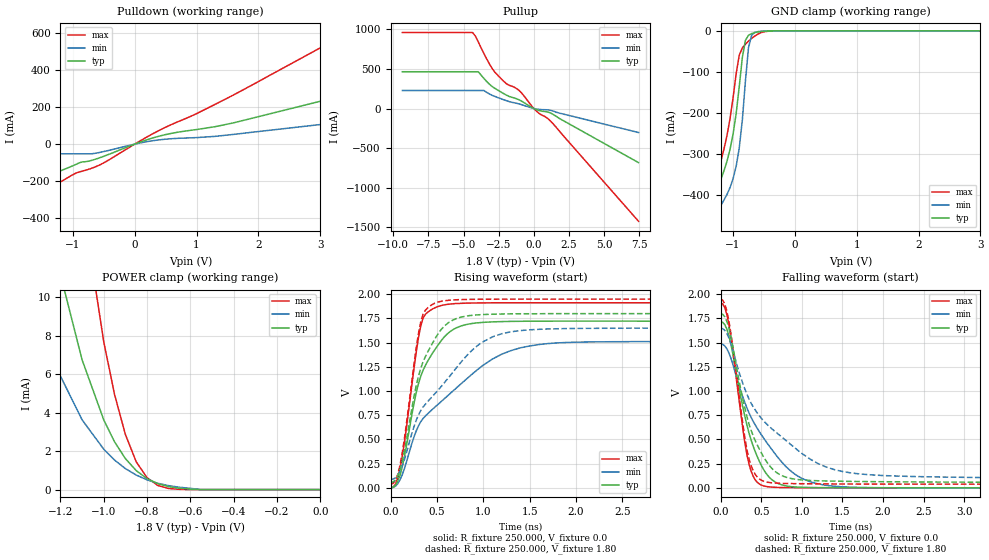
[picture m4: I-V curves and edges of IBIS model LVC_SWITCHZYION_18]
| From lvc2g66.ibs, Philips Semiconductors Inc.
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|   Model LVC_SWITCHZYION_18
[Model]   LVC_SWITCHZYION_18
Model_type   I/O
Polarity   Non-Inverting
Enable   Active-High
Vinl  =  0.63V
Vinh  =  1.17V
Vmeas =  0.90V
Cref  =  30.0pF
Rref  =  1.0k
Vref  =  0.0V
C_comp   7.87pF   4.23pF   10.52pF
[Model Spec]
| Note: The input and output voltage ratings may be exceeded if the input and
|   output current ratings are observed (please refer to the data sheet)
|   Subparameter   typ   min   max
| Thresholds
Vinh   1.17   1.0725   1.2675
Vinl   0.63   0.5775   0.6825
| Overshoot
S_overshoot_high   6.5   6.5   6.5   | Static overshoot
S_overshoot_low   -0.5   -0.5   -0.5
D_overshoot_high   7.2   7.2   7.2   | Dynamic overshoot
D_overshoot_low   -0.95   -0.9   -1.0
D_overshoot_time   3n   3n   3n
| Timing Thresholds
Vmeas   0.9   0.825   0.975
|Ambient temperature:   25   85   -40
[Temperature Range]   25   85   -40
[Voltage Range]   1.80V   1.65V   1.95V
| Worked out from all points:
|   slope of the pulldown table from 0 to 0.27 V, typ, clamps not added: 8.71 ohm
|   slope of the pullup table from 0 to 0.27 V, typ, clamps not added: 13.9 ohm
|   GND clamp passes 1 mA (typ) near -0.50 V on its own axis
|   POWER clamp passes 1 mA (typ) near -0.85 V on its own axis
|   rising waveform, R_fixture 250.000, V_fixture 0.0: 20-80 % time 288ps typ, 734ps min, 161ps max; typ from 0 V to 1.72 V
|   rising waveform, R_fixture 250.000, V_fixture 1.80: 20-80 % time 273ps typ, 613ps min, 161ps max; typ from 0.056 V to 1.8 V
|   falling waveform, R_fixture 250.000, V_fixture 0.0: 20-80 % time 289ps typ, 542ps min, 185ps max; typ from 1.72 V to 0 V
|   falling waveform, R_fixture 250.000, V_fixture 1.80: 20-80 % time 322ps typ, 754ps min, 188ps max; typ from 1.8 V to 0.056 V
|Process Range   nominal   slow   fast
[Pulldown]
| voltage   I(typ)   I(min)   I(max)
-5.5V     -260.6mA   -52.23mA   -443.6mA
-2.3V     -260.6mA   -52.23mA   -443.6mA
-2.1V     -260.6mA   -52.23mA   -388.5mA
-1.05V    -124.3mA   -52.23mA   -175mA
-700mV    -88.32mA   -52.23mA   -131.2mA
400mV     43.47mA    23.26mA    74.9mA
1.6V      115.3mA    52.71mA    266.4mA
3.4V      265.4mA    121.1mA    593.8mA
3.7V      290.4mA    132.4mA    648.5mA
7.6V      615.6mA    279.8mA    1.359A
7.9V      640.6mA    291.2mA    1.414A
11V       899.1mA    408.3mA    1.978A
[Pullup]
| voltage   I(typ)   I(min)   I(max)
-9.35V    464.7mA    227.8mA    959.7mA
-4.35V    464.7mA    227.8mA    959.7mA
-4.15V    464.7mA    227.8mA    913.3mA
-3.95V    464.7mA    227.8mA    840.9mA
-3.55V    380.5mA    227.8mA    695.7mA
-3.15V    306mA      183.2mA    560.8mA
-2.75V    252.5mA    151.3mA    454.6mA
-1.95V    169.5mA    98.93mA    313.6mA
-950mV    101.1mA    53.15mA    212.3mA
200mV     -15.4mA    -7.129mA   -36.04mA
1.2V      -57.74mA   -23.05mA   -160.2mA
7.45V     -683.5mA   -303.4mA   -1.425A
[GND_clamp]
| voltage   I(typ)   I(min)   I(max)
-5.5V     -5.537A    -5.177A    -6.202A
-1.4V     -516.4mA   -571.8mA   -481.4mA
-1.35V    -470.1mA   -525.9mA   -434.4mA
-1.3V     -425.7mA   -482.2mA   -389mA
-1.1V     -319.2mA   -399.7mA   -256.6mA
-950mV    -201.8mA   -330.3mA   -104.7mA
-900mV    -136.1mA   -285.8mA   -59.42mA
-850mV    -65.02mA   -217.8mA   -41.68mA
-800mV    -23.2mA    -121.8mA   -32.63mA
-750mV    -10.8mA    -40.76mA   -25.13mA
-650mV    -4.467mA   -3.964mA   -12.76mA
5.5V      399.8pA    5.379nA    29.89pA
[POWER_clamp]
| voltage   I(typ)   I(min)   I(max)
-9.35V    7.563A     7.588A     7.618A
-1.4V     22.03mA    13.31mA    49.14mA
-1.25V    13.39mA    7.034mA    30.13mA
-1.1V     6.742mA    3.623mA    15.03mA
-1V       3.622mA    2.099mA    7.68mA
-950mV    2.481mA    1.535mA    4.939mA
-900mV    1.612mA    1.092mA    2.864mA
-850mV    987.7uA    755.2uA    1.448mA
-800mV    570.3uA    507.7uA    617.9uA
-750mV    307.3uA    328.4uA    212.9uA
-650mV    69.44uA    121.7uA    13.64uA
0V        0A         0A         0A
[Ramp]
| variable   typ   min   max
dV/dt_r   1.032V/287.683ps   903.161mV/733.821ps   1.147V/161.267ps
dV/dt_f   1.047V/321.661ps   936.914mV/753.761ps   1.147V/187.763ps
R_load = 250.000
[Rising Waveform]
R_fixture   = 250.000
V_fixture   = 0.0
V_fixture_min = 0.0
V_fixture_max = 0.0
| time   V(typ)   V(min)   V(max)
0s        0V         -83.19pV   0V
75ps      61.63mV    39.82mV    93.82mV
125ps     213.7mV    133.3mV    316.6mV
325ps     1.152V     682.8mV    1.672V
375ps     1.264V     741.9mV    1.793V
550ps     1.526V     895.6mV    1.885V
750ps     1.669V     1.067V     1.906V
1.1ns     1.715V     1.332V     1.912V
1.7ns     1.722V     1.491V     1.912V
8.8ns     1.719V     1.505V     1.911V
[Rising Waveform]
R_fixture   = 250.000
V_fixture   = 1.80
V_fixture_min = 1.65
V_fixture_max = 1.95
| time   V(typ)   V(min)   V(max)
0s        55.63mV    86.4mV     38.05mV
50ps      78.77mV    102.3mV    72.84mV
100ps     182.6mV    167.9mV    227.6mV
325ps     1.234V     798.3mV    1.714V
375ps     1.355V     863.8mV    1.835V
525ps     1.61V      1.024V     1.923V
700ps     1.746V     1.229V     1.943V
975ps     1.79V      1.496V     1.949V
1.5ns     1.799V     1.633V     1.95V
8.8ns     1.8V       1.651V     1.95V
[Falling Waveform]
R_fixture   = 250.000
V_fixture   = 0.0
V_fixture_min = 0.0
V_fixture_max = 0.0
| time   V(typ)   V(min)   V(max)
0s        1.717V     1.488V     1.911V
100ps     1.575V     1.396V     1.69V
275ps     826.1mV    933.7mV    597.3mV
350ps     562.6mV    772mV      241.1mV
425ps     375.6mV    650.5mV    83.46mV
525ps     194.2mV    518.5mV    21.16mV
675ps     58.4mV     346.1mV    5.405mV
925ps     8.48mV     135.3mV    2.275mV
1.4ns     1.433mV    16.51mV    934.1uV
8.8ns     -668.1nV   -51.5uV    -38.13nV
[Falling Waveform]
R_fixture   = 250.000
V_fixture   = 1.80
V_fixture_min = 1.65
V_fixture_max = 1.95
| time   V(typ)   V(min)   V(max)
0s        1.8V       1.65V      1.95V
100ps     1.654V     1.551V     1.728V
275ps     907.3mV    1.073V     647.8mV
350ps     655.2mV    915.9mV    294.8mV
425ps     488.9mV    805mV      140.2mV
550ps     290.2mV    672.6mV    63.04mV
775ps     118.8mV    509.7mV    45.85mV
1.2ns     73.28mV    250.8mV    41.18mV
1.8ns     64.86mV    137.4mV    39.08mV
8.8ns     55.66mV    88.48mV    38.05mV
